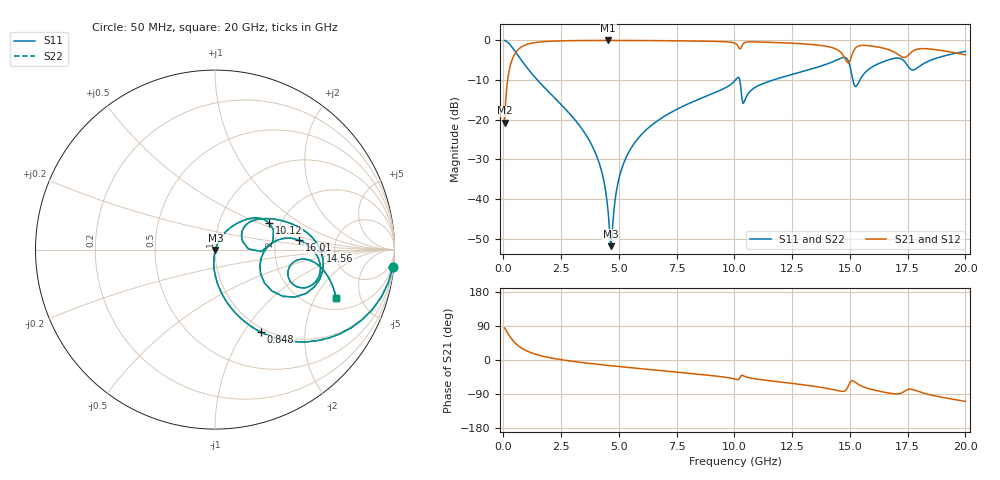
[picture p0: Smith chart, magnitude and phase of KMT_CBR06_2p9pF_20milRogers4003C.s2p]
! Data measured by Modelithics Inc. support@modelithics.com 813-866-6335
! KEMET CBR0603 2.9pF, Pad Width= 0.851mm, Pad Length= 0.64mm, Pad Gap= 0.62mm, 20mil Rogers 4003C substrate Data, January 2022
# hz S ma R 50
! 2 Port Network Data from SP1.SP block
! freq  magS11  angS11  magS21  angS21  magS12  angS12  magS22  angS22
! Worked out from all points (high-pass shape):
!   401 points, 50 MHz to 20 GHz, reference 50 ohm
!   highest |S21| = -0.02 dB at 4.539 GHz (marker M1); lowest = -20.7 dB at 50 MHz (marker M2)
!   |S21| within 3 dB of the highest: 536.1 MHz to 14.6 GHz (14.07 GHz wide, 186 % of centre); 15.13 GHz to 16.94 GHz (1.811 GHz wide, 11.3 % of centre)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
!   lowest |S11| = -51.8 dB at 4.638 GHz (marker M3), VSWR 1.01, Z = 50.2 - j0.142 ohm
!   |S11| at or under -10 dB: 1.472 GHz to 10.05 GHz (8.573 GHz wide, 149 % of centre); 10.23 GHz to 11.67 GHz (1.443 GHz wide, 13.2 % of centre); 15.13 GHz to 15.43 GHz (301.1 MHz wide, 1.97 % of centre)
!   |S22| runs from -51.8 to 0.0 dB; largest |S21 - S12| = 0
!   S11 on the Smith chart (normalised r, x): 50 MHz: 1, -21; 848 MHz: 0.95, -1.20; 10.12 GHz: 1.74, +0.58; 14.56 GHz: 3.86, -0.06; 16.01 GHz: 2.72, +0.37; 20 GHz: 2.66, -3.02
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5e7  0.9958 -5.4  0.09175 84.6  0.09175 84.6  0.9958 -5.4
3.4925e8  0.8392 -34.0  0.543 55.9  0.543 55.9  0.8392 -34.0
8.48e8  0.5264 -60.9  0.8491 29.0  0.8491 29.0  0.5264 -60.9
1.695875e9  0.2691 -79.6  0.9616 10.1  0.9616 10.1  0.2691 -79.6
3.391625e9  0.07719 -95.1  0.9948 -6.6  0.9948 -6.6  0.07719 -95.1
4.189625e9  0.02586 -97.0  0.9972 -12.1  0.9972 -12.1  0.02586 -97.0
4.53875e9  0.006626 -83.2  0.9974 -14.4  0.9974 -14.4  0.006626 -83.2
4.6385e9  0.002558 -33.5  0.9974 -15.0  0.9974 -15.0  0.002558 -33.5
4.987625e9  0.01752 64.5  0.9971 -17.2  0.9971 -17.2  0.01752 64.5
5.286875e9  0.03235 66.4  0.9967 -19.0  0.9967 -19.0  0.03235 66.4
6.73325e9  0.09995 60.7  0.9917 -27.5  0.9917 -27.5  0.09995 60.7
1.0025e10  0.3111 33.8  0.9183 -50.2  0.9183 -50.2  0.3111 33.8
1.012475e10  0.3367 26.0  0.8725 -51.7  0.8725 -51.7  0.3367 26.0
1.0424e10  0.1677 28.1  0.9316 -42.6  0.9316 -42.6  0.1677 28.1
1.336662e10  0.4391 19.8  0.8861 -68.7  0.8861 -68.7  0.4391 19.8
1.456362e10  0.5885 -0.5  0.7242 -81.9  0.7242 -81.9  0.5885 -0.5
1.496262e10  0.5187 -30.6  0.5251 -64.2  0.5251 -64.2  0.5187 -30.6
1.526188e10  0.2619 -9.8  0.8115 -60.0  0.8115 -60.0  0.2619 -9.8
1.601e10  0.4712 6.4  0.8423 -78.7  0.8423 -78.7  0.4712 6.4
1.670825e10  0.5723 -3.9  0.758 -87.5  0.758 -87.5  0.5723 -3.9
1.770575e10  0.4239 -16.2  0.7253 -77.7  0.7253 -77.7  0.4239 -16.2
2e10  0.726 -21.6  0.6567 -109.2  0.6567 -109.2  0.726 -21.6
